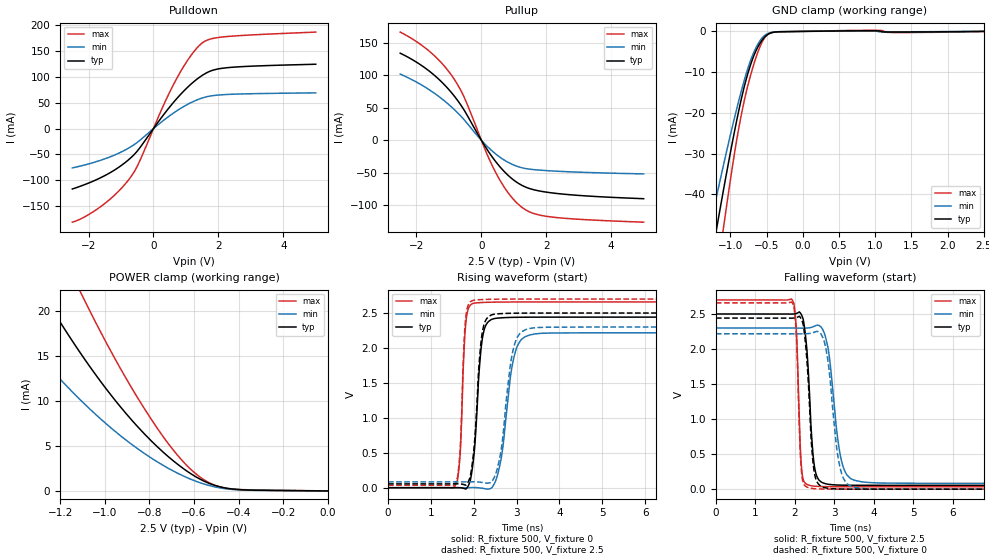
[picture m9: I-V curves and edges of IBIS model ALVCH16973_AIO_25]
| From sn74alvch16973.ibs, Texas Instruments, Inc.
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[Model]   ALVCH16973_AIO_25
Model_type  I/O
Vinl=0.7
Vinh=1.7
Enable   Active-Low
Vref =   0
Rref =   500
Cref =   30p
Vmeas =   1.25
| variable   typ   min   max
C_comp   3.43pF   3.01pF   3.69pF
| C_pullup   4.62pF   3.59pF   5.34pF
| C_pulldown   4.70pF   3.22pF   6.51pF
| C_tri-state   3.43pF   3.01pF   3.69pF
[Temperature Range]   40   100   -40
| Ambient temperature   25   85   -40
[Voltage range]   2.5   2.3   2.7
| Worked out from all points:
|   slope of the pulldown table from 0 to 0.375 V, typ, clamps not added: 11.7 ohm
|   slope of the pullup table from 0 to 0.375 V, typ, clamps not added: 13.2 ohm
|   GND clamp passes 1 mA (typ) near -0.50 V on its own axis
|   POWER clamp passes 1 mA (typ) near -0.55 V on its own axis
|   rising waveform, R_fixture 500, V_fixture 0: 20-80 % time 156ps typ, 258ps min, 99.6ps max; typ from 0 V to 2.44 V
|   falling waveform, R_fixture 500, V_fixture 2.5: 20-80 % time 151ps typ, 258ps min, 94.2ps max; typ from 2.5 V to 0.055 V
|   rising waveform, R_fixture 500, V_fixture 2.5: 20-80 % time 155ps typ, 246ps min, 94.7ps max; typ from 0.055 V to 2.5 V
|   falling waveform, R_fixture 500, V_fixture 0: 20-80 % time 154ps typ, 246ps min, 92.6ps max; typ from 2.44 V to 0 V
[GND Clamp]
| ALVCH16973_AIO_25
|   Voltage   I(typ)   I(min)   I(max)
-2.5V     -196mA     -160.6mA   -242mA
-1.295V   -59.12mA   -49.03mA   -73.93mA
-1.26V    -55.47mA   -46.1mA    -69.3mA
-1.19V    -48.28mA   -40.32mA   -60.15mA
-1.1V     -39.27mA   -33.09mA   -48.64mA
-1.06V    -35.37mA   -29.95mA   -43.64mA
-905mV    -21.13mA   -18.41mA   -25.74mA
-795mV    -12.6mA    -11.15mA   -15.87mA
-635mV    -4.298mA   -3.567mA   -5.766mA
-500mV    -955.7uA   -674.7uA   -1.004mA
535mV     116.6uA    68.81uA    193.2uA
2.5V      837.7pA    30.92uA    -60.81uA
[POWER Clamp]
| ALVCH16973_AIO_25
|   Voltage   I(typ)   I(min)   I(max)
-2.5V     88.63mA    62.79mA    110mA
-1.52V    32.72mA    21.99mA    45.11mA
-1.495V   31.53mA    21.17mA    43.61mA
-1.27V    21.55mA    14.31mA    30.61mA
-1.095V   14.79mA    9.751mA    21.37mA
-935mV    9.486mA    6.232mA    13.81mA
-790mV    5.511mA    3.621mA    7.886mA
-670mV    2.89mA     1.921mA    3.844mA
-580mV    1.401mA    968.8uA    1.666mA
-520mV    722.5uA    523.2uA    765.4uA
-445mV    264.7uA    204.2uA    262.3uA
-31.15fV  837.7pA    2.097nA    92.36pA
[Pulldown]
| ALVCH16973_AIO_25
|   Voltage   I(typ)   I(min)   I(max)
-2.5V     -116.7mA   -75.94mA   -180.9mA
-1.52V    -91.51mA   -58.89mA   -145.8mA
-1.075V   -74.92mA   -47.63mA   -121mA
-700mV    -56.45mA   -35.17mA   -93.45mA
-455mV    -39.93mA   -24.42mA   -66.85mA
265mV     22.95mA    13.69mA    39.02mA
675mV     54.98mA    32.57mA    92.13mA
1.115V    83.7mA     48.99mA    137.9mA
1.495V    102.6mA    59.02mA    165.3mA
1.83V     112.9mA    63.78mA    174.4mA
2.275V    117.8mA    66.07mA    178.1mA
5V        124.5mA    69.16mA    186.7mA
[Pullup]
| ALVCH16973_AIO_25
|   Voltage   I(typ)   I(min)   I(max)
-2.5V     134mA      101.9mA    166.5mA
-1.585V   105.6mA    77.05mA    136.2mA
-1.21V    89.01mA    63.51mA    118mA
-890mV    71.4mA     49.86mA    97.84mA
-525mV    45.85mA    31.23mA    65.64mA
135mV     -10.99mA   -7.123mA   -16.78mA
455mV     -33.71mA   -21.58mA   -50.91mA
840mV     -54.72mA   -34.35mA   -81.84mA
1.235V    -68.97mA   -42.11mA   -102.6mA
1.6V      -75.94mA   -45.08mA   -112.5mA
2.145V    -80.8mA    -47.11mA   -118mA
5V        -89.91mA   -51.75mA   -126mA
[Ramp]
| ALVCH16973_AIO_25
| variable   typ   min   max
dV/dt_r   1.48/1.60E-10   1.34/2.69E-10   1.60/1.01E-10
dV/dt_f   1.48/1.58E-10   1.35/2.70E-10   1.61/1.01E-10
R_load = 500
[Rising Waveform]
| ALVCH16973_AIO_25
R_fixture =   500
C_fixture =   0
L_fixture =   0
V_fixture =   0
V_fixture_min = 0
V_fixture_max = 0
|   Time   V(typ)   V(min)   V(max)
0s        6.767nV    30.52nV    187.6pV
1.58ns    886.7uV    28.15uV    45.4mV
1.685ns   -909.1uV   165.6uV    499.8mV
1.815ns   -19.03mV   553.7uV    2.358V
2.03ns    652mV      1.958mV    2.643V
2.285ns   2.329V     -17.9mV    2.653V
2.605ns   2.43V      309mV      2.657V
2.985ns   2.439V     1.974V     2.658V
3.435ns   2.441V     2.202V     2.659V
29.99ns   2.441V     2.217V     2.659V
[Falling Waveform]
| ALVCH16973_AIO_25
R_fixture =   500
C_fixture =   0
L_fixture =   0
V_fixture =   2.5
V_fixture_min = 2.3
V_fixture_max = 2.7
|   Time   V(typ)   V(min)   V(max)
0s        2.5V       2.3V       2.7V
1.945ns   2.499V     2.299V     2.686V
2.03ns    2.506V     2.299V     2.324V
2.175ns   2.475V     2.298V     253mV
2.305ns   1.968V     2.299V     68.14mV
2.44ns    614.8mV    2.313V     46.16mV
2.815ns   72.75mV    2.074V     36.28mV
3.21ns    56.97mV    336.3mV    35.06mV
3.7ns     55.12mV    104.1mV    34.82mV
29.99ns   54.78mV    83.35mV    34.78mV
[Rising Waveform]
| ALVCH16973_AIO_25
R_fixture =   500
C_fixture =   0
L_fixture =   0
V_fixture =   2.5
V_fixture_min = 2.3
V_fixture_max = 2.7
|   Time   V(typ)   V(min)   V(max)
0s        54.78mV    83.35mV    34.78mV
1.58ns    55.54mV    83.39mV    81.83mV
1.685ns   53.64mV    83.51mV    558.7mV
1.815ns   36.41mV    83.82mV    2.447V
2.025ns   707.8mV    84.8mV     2.685V
2.26ns    2.372V     68.68mV    2.695V
2.585ns   2.49V      363.5mV    2.699V
2.965ns   2.498V     2.075V     2.7V
3.39ns    2.499V     2.287V     2.7V
29.99ns   2.5V       2.3V       2.7V
[Falling Waveform]
| ALVCH16973_AIO_25
R_fixture =   500
C_fixture =   0
L_fixture =   0
V_fixture =   0
V_fixture_min = 0
V_fixture_max = 0
|   Time   V(typ)   V(min)   V(max)
0s        2.441V     2.217V     2.659V
1.94ns    2.441V     2.217V     2.648V
2.03ns    2.447V     2.217V     2.257V
2.175ns   2.406V     2.216V     195.1mV
2.295ns   1.894V     2.218V     32.99mV
2.425ns   594mV      2.228V     11.48mV
2.77ns    19.38mV    2.04V      1.692mV
3.18ns    1.873mV    224.7mV    293uV
3.61ns    353.7uV    18.05mV    49.93uV
29.99ns   32.12nV    70.36nV    -1.618nV
